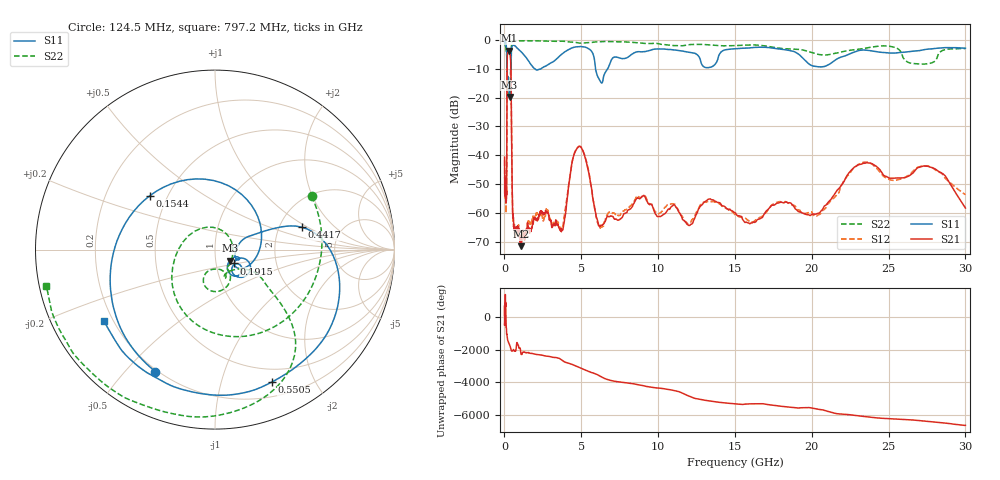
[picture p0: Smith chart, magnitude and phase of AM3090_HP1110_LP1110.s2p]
! Date/Time: Thu, Feb 28, 2019 2:09 PM
! Network Analyzer: Agilent Technologies E8364B Rev: A.07.50.67
! Sweep from 0.010 to 30.000 GHz, 1601 Points, Sweep Type: LOG
! Power Supply: 5.023 V, 0.002 A
# Hz S DB R 50
!freq MagS11 AngS11 MagS21 AngS21 MagS12 AngS12 MagS22 AngS22
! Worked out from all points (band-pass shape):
!   1601 points, 10 MHz to 30 GHz, reference 50 ohm
!   highest |S21| = -3.74 dB at 273.2 MHz (marker M1); lowest = -71.5 dB at 1.098 GHz (marker M2)
!   |S21| within 3 dB of the highest: 178.5 MHz to 401.3 MHz (222.8 MHz wide, 76.8 % of centre)
!   lowest |S11| = -19.8 dB at 330.4 MHz (marker M3), VSWR 1.23, Z = 58.4 - j7.32 ohm
!   |S11| at or under -10 dB: 166 MHz to 423.4 MHz (257.4 MHz wide, 87.4 % of centre); 1.973 GHz to 2.382 GHz (409.6 MHz wide, 18.8 % of centre); 5.93 GHz to 6.72 GHz (789.7 MHz wide, 12.5 % of centre)
!   |S22| runs from -20.0 to -0.2 dB; largest |S21 - S12| = 0.016
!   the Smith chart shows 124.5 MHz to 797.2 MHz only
!   S11 on the Smith chart (normalised r, x): 124.5 MHz: 0.19, -0.61; 154.4 MHz: 0.40, +0.31; 191.5 MHz: 1.22, -0.19; 441.7 MHz: 2.65, +0.88; 550.5 MHz: 0.35, -1.46; 797.2 MHz: 0.17, -0.29
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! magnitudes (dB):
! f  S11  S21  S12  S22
! 10 MHz  -0.3  -40.6  -41.7  -0.7
! 38.04 MHz  -0.3  -51.0  -49.6  -1.4
! 124.5 MHz  -2.4  -54.9  -53.6  -4.2
! 144.7 MHz  -4.5  -49.1  -47.9  -5.3
! 154.4 MHz  -6.5  -31.7  -31.6  -7.3
! 169.8 MHz  -11.2  -10.3  -10.3  -19.3
! 191.5 MHz  -17.6  -5.0  -5.0  -18.1
! 273.2 MHz  -15.5  -3.7  -3.7  -18.3
! 330.4 MHz  -19.8  -4.1  -4.1  -16.6
! 403.6 MHz  -13.9  -7.0  -7.0  -9.3
! 441.7 MHz  -6.0  -20.4  -20.3  -3.0
! 550.5 MHz  -1.9  -60.6  -62.6  -0.4
! 797.2 MHz  -2.7  -66.1  -65.1  -0.3
! 1.098 GHz  -4.2  -71.5  -68.2  -0.3
! 2.084 GHz  -10.4  -62.5  -60.7  -0.3
! 3.723 GHz  -4.9  -65.7  -65.0  -0.4
! 4.854 GHz  -2.4  -36.9  -36.9  -1.1
! 6.202 GHz  -14.0  -64.8  -65.2  -0.6
! 7.926 GHz  -6.3  -59.9  -58.8  -0.7
! 20.1 GHz  -9.1  -60.3  -60.8  -4.5
! 23.48 GHz  -3.5  -42.7  -42.4  -2.9
! 30 GHz  -2.9  -58.3  -53.6  -3.0
